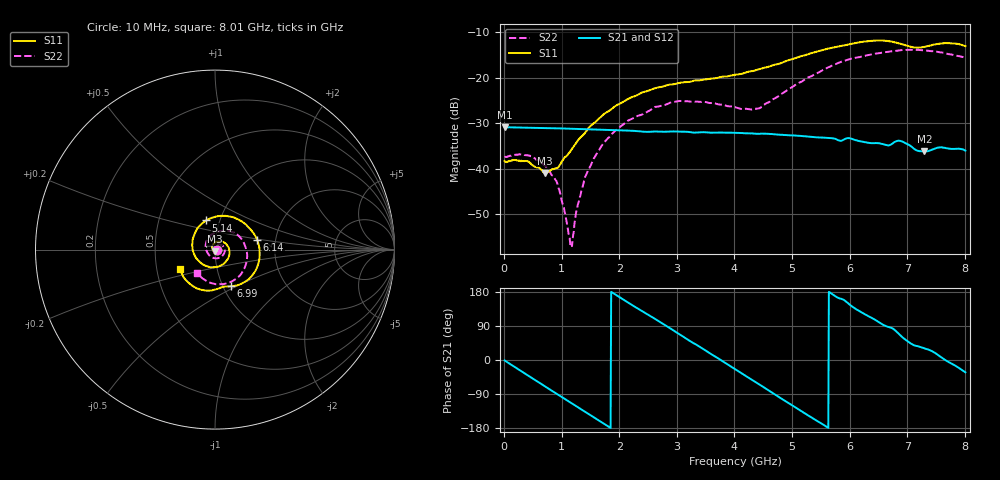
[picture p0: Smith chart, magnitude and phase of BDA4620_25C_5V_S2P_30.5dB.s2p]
!Agilent Technologies,E5071B,MY42404982,A.09.10
!Date: Wed May 06 09:05:06 2026
!Data & Calibration Information:
!Freq	S11:SOLT2(ON)	S21:SOLT2(ON)	S12:SOLT2(ON)	S22:SOLT2(ON)
# Hz S RI R 50
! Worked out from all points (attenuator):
!   801 points, 10 MHz to 8.01 GHz, reference 50 ohm
!   highest |S21| = -30.88 dB at 10 MHz (marker M1); lowest = -36.2 dB at 7.3 GHz (marker M2)
!   lowest |S11| = -40.9 dB at 710 MHz (marker M3), VSWR 1.02, Z = 49.9 - j0.892 ohm
!   |S11| at or under -10 dB: start of sweep to end of sweep
!   |S22| runs from -56.9 to -13.9 dB; largest |S21 - S12| = 0.00019
!   S11 on the Smith chart (normalised r, x): 10 MHz: 1.02, -0.00; 5.14 GHz: 0.86, +0.29; 6.14 GHz: 1.60, +0.18; 6.99 GHz: 1.09, -0.47; 8.01 GHz: 0.66, -0.15
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1e7  0.0121 -0.000736  0.0286 -0.000572  0.0286 -0.00058  0.0135 -0.00044
4.3e8  0.00843 -0.00849  0.0208 -0.019  0.0209 -0.0191  0.0132 -0.00472
7.1e8  -0.000911 -0.00894  0.00976 -0.0262  0.00979 -0.0263  0.00847 -0.00667
9.4e8  -0.0094 -0.00433  -0.000916 -0.0277  -0.000969 -0.0278  0.00334 -0.00534
1.16e9  -0.0148 0.00563  -0.0108 -0.0253  -0.0109 -0.0253  -0.00123 -0.00074
1.19e9  -0.0153 0.00726  -0.0121 -0.0247  -0.0121 -0.0247  -0.00165 0.000145
1.35e9  -0.0155 0.0166  -0.018 -0.0204  -0.0181 -0.0204  -0.00318 0.00494
1.53e9  -0.0114 0.0283  -0.023 -0.0141  -0.0231 -0.0141  -0.00294 0.0114
1.77e9  0.00174 0.0411  -0.0264 -0.00392  -0.0265 -0.0039  0.00119 0.0204
2.14e9  0.0346 0.0459  -0.0234 0.012  -0.0234 0.012  0.0169 0.0287
2.68e9  0.0777 0.00678  -0.00563 0.0249  -0.00561 0.025  0.0441 0.0191
3.08e9  0.0738 -0.0478  0.011 0.023  0.011 0.023  0.0549 -0.00754
4.01e9  -0.0687 -0.082  0.0226 -0.0101  0.0226 -0.0101  -0.0105 -0.0461
4.43e9  -0.1235 -0.0051  0.0106 -0.0217  0.0105 -0.0218  -0.0446 -0.0113
5.14e9  -0.0507 0.1622  -0.0156 -0.0168  -0.0156 -0.0168  -0.0124 0.0877
5.35e9  0.0116 0.1857  -0.0199 -0.0102  -0.0199 -0.0102  0.0232 0.1019
6.14e9  0.2355 0.0521  -0.0135 0.0152  -0.0135 0.0152  0.1627 0.0333
6.68e9  0.1918 -0.1609  0.000948 0.018  0.000938 0.0181  0.1697 -0.0894
6.99e9  0.0908 -0.2039  0.0117 0.0147  0.0118 0.0147  0.1261 -0.156
7.3e9  0.0238 -0.2154  0.0133 0.00786  0.0134 0.00792  0.0536 -0.191
7.65e9  -0.096 -0.2176  0.017 0.000277  0.017 0.000217  -0.0323 -0.1822
8.01e9  -0.1927 -0.1068  0.0133 -0.00851  0.0135 -0.00854  -0.1025 -0.1282
